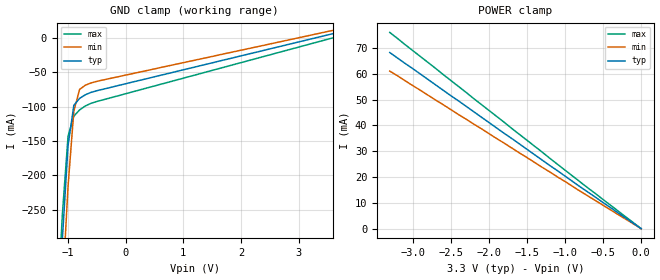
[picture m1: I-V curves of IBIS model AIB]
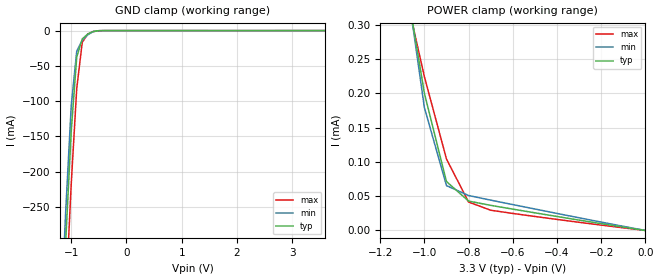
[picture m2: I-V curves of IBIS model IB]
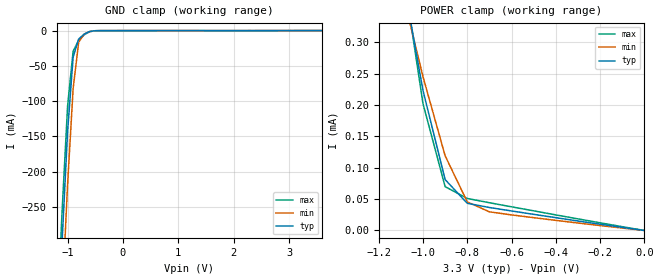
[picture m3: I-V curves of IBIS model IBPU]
|   Texas Instruments Incorporated
|   DVI group
|   IBIS Model for TFP401 Rev.st0n1
|   100 pin PowerPAD Package
[IBIS Ver]   4.0
[Comment char]   |_char
[File name]   tfp401n_st0.ibs
[File Rev]   1.0
[Date]   10/25/2002
[Source]   File originated at Texas Instruments Incorporated.
   Bus Solutions Department. All data based on SPICE
   simulation.
[Notes]   File created by Ellen Yeh.
   PIN #3 (ST) set to low.
|Revision log: 1.0, 10/25/2002 Original release
[Disclaimer]
(C) Copyright Texas Instruments Incorporated 2002
   All rights reserved
  Texas Instruments Incorporated hereby grants the user of this IBIS
model a non-exclusive, nontransferable license to use this IBIS model
under the following terms.  Before using this IBIS model, the user
should read this license.  If the user does not accept these terms,
the IBIS model should be returned to Texas Instruments within 30 days.
  The user is granted this license only to use the IBIS model and
is not granted rights to sell, load, rent, lease or license the IBIS
model in whole or in part, or in modified form to anyone other than
user.  User may modify the IBIS model to suit its specific applications
but rights to derivative works and such modifications shall belong to
Texas Instruments.
  This IBIS model is provided on an "AS IS" basis and Texas Instruments
makes absolutely no warranty with respect to the information contained
herein.  TEXAS INSTRUMENTS DISCLAIMS AND CUSTOMER WAIVES ALL WARRANTIES,
EXPRESS OR IMPLIED, INCLUDING WARRANTIES OF MERCHANTABILITY OR FITNESS
FOR A PARTICULAR PURPOSE. The entire risk as to quality and performance
is with the Customer. ACCORDINGLY, IN NO EVENT SHALL THE COMPANY BE LIABLE
FOR ANY DAMAGES, WHETHER IN CONTRACT OR TORT,INCLUDING ANY LOST PROFITS
OR OTHER INCIDENTAL, CONSEQUENTIAL, EXEMPLARY, OR PUNITIVE DAMAGES ARISING
OUT OF THE USE OR APPLICATION OF THE IBIS model provided in this package.
Further, Texas Instruments reserves the right to discontinue or make changes
without notice to any product herein to improve reliability, function, or
design. Texas Instruments does not convey any license under patent rights
or any other intellectual property rights, including those of third parties.
IBIS Open Forum disclaims all warranties. See DISCLAIM.TXT
in vhdl.org:/pub/IBIS/models for the full disclaimer.
[Copyright]   Copyright 2002, Texas Instruments, All Rights Reserved
[Component]   TFP401
[Manufacturer]  Texas Instruments Incorporated
[Package]
|   typ   min   max
R_pkg   0.051   0.049   0.054
L_pkg   2.9nH   2.7nH   3.2nH
C_pkg   0.44pF   0.36pF   0.5pF
[Pin]   signal_name   model_name   R_pin   L_pin   C_pin
1   DFO   IOBOD
2   PDZ   IBPU
3   ST   IB
4   PIXS   IB
5   GND   GND
6   DVDD   POWER
7   STAG   IB
8   SCDT   IOB
9   PDOZ   IBPU
10   QE0   OB
11   QE1   OB
12   QE2   OB
13   QE3   OB
14   QE4   OB
15   QE5   OB
16   QE6   OB
17   QE7   OB
18   OVDD   POWER
19   OGND   GND
20   QE8   OB
21   QE9   OB
22   QE10   OB
23   QE11   OB
24   QE12   OB
25   QE13   OB
26   QE14   OB
27   QE15   OB
28   OGND   GND
29   OVDD   POWER
30   QE16   OB
31   QE17   OB
32   QE18   OB
33   QE19   OB
34   QE20   OB
35   QE21   OB
36   QE22   OB
37   QE23   OB
38   DVDD   POWER
39   GND   GND
40   CTL1   IOB
41   CTL2   IOB
42   CTL3   IOB
43   OVDD   POWER
44   ODCK   OB2
45   OGND   GND
46   DE   OB
47   VSYNC   OB
48   HSYNC   OB
49   QO0   OB
50   QO1   OB
51   QO2   OB
52   QO3   OB
53   QO4   OB
54   QO5   OB
55   QO6   OB
56   QO7   OB
57   OVDD   POWER
58   OGND   GND
59   QO8   OB
60   QO9   OB
61   QO10   OB
62   QO11   OB
63   QO12   OB
64   QO13   OB
65   QO14   OB
66   QO15   OB
67   DVDD   POWER
68   GND   GND
69   QO16   OB
70   QO17   OB
71   QO18   OB
72   QO19   OB
73   QO20   OB
74   QO21   OB
75   QO22   OB
76   OGND   GND
77   QO23   OB
78   OVDD   POWER
79   AGND   GND
80   RX2+   AIB
81   RX2-   AIB
82   AVDD   POWER
83   AGND   GND
84   AVDD   POWER
85   RX1+   AIB
86   RX1-   AIB
87   AGND   GND
88   AVDD   POWER
89   AGND   GND
90   RX0+   AIB
91   RX0-   AIB
92   AGND   GND
93   RXC+   AIB
94   RXC-   AIB
95   AVDD   POWER
96   EXT_RES   AIB
97   PVDD   POWER
98   PGND   GND
99   RSVD   IBPU
100   OCK_INV   IB
| Models and submodels in the file (7): AIB (Input), IB (Input), IBPU (Input), IOB (I/O), IOBOD (I/O_open_sink), OB (3-state), OB2 (3-state)
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|   INPUT  MODEL
[Model]   AIB
Model_type   Input
Vinl = 2.85
Vinh = 3.0
| variable   typ   min   max
C_comp   2pF   NA   NA
|   typ   min   max
[Temperature Range]   25.0   70   0
[Voltage range]   3.3V   3.0V   3.6V
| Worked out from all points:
|   POWER clamp passes 1 mA (typ) near -0.05 V on its own axis
[GND_clamp]
|Voltage   I(typ)   I(min)   I(max)
-3.6V     -5.13A     -5.2A      -5.09A
-1.2V     -463mA     -543mA     -422mA
-1.1V     -295mA     -371mA     -259mA
-1V       -157mA     -216mA     -143mA
-900mV    -98.3mA    -107mA     -114mA
-800mV    -88.2mA    -75.2mA    -105mA
-700mV    -82.9mA    -69mA      -99.2mA
-500mV    -77mA      -63.4mA    -92.7mA
3.6V      6.08mA     10.9mA     8.48pA
[Power_clamp]
|Note that the [Power_clamp] voltage table is referenced to Vcc
|and is calculated using Vtable=Vcc-Vmeasured.
|Voltage   I(typ)   I(min)   I(max)
-3.3V     68.3mA     61.1mA     76.1mA
-1.2V     24.5mA     22mA       27.3mA
-800mV    16.2mA     14.5mA     18.1mA
0V        10.1pA     47.9pA     8.48pA
|   INPUT  MODEL
[Model]   IB
Model_type   Input
Vinl = 0.8
Vinh = 2.0
| variable   typ   min   max
C_comp   2pF   NA   NA
|   typ   min   max
[Temperature Range]   25.0   70   0
[Voltage range]   3.3V   3.0V   3.6V
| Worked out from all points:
|   GND clamp passes 1 mA (typ) near -0.58 V on its own axis
|   POWER clamp passes 1 mA (typ) near -1.37 V on its own axis
[GND_clamp]
|Voltage   I(typ)   I(min)   I(max)
-3.6V     -5.15A     -5.11A     -5.23A
-1.2V     -475mA     -430mA     -560mA
-1.1V     -300mA     -257mA     -383mA
-1V       -143mA     -107mA     -218mA
-900mV    -37.5mA    -29.1mA    -82.2mA
-800mV    -11.8mA    -13.8mA    -16.6mA
-700mV    -4.88mA    -5.9mA     -4.87mA
-600mV    -1.21mA    -1.39mA    -1.38mA
-500mV    -134uA     -137uA     -206uA
3.6V      15.1uA     34.3pA     24.8uA
[Power_clamp]
|Note that the [Power_clamp] voltage table is referenced to Vcc
|and is calculated using Vtable=Vcc-Vmeasured.
|Voltage   I(typ)   I(min)   I(max)
-3.3V     5.59mA     6.88mA     4.02mA
-1.1V     393uA      406uA      367uA
-1V       200uA      179uA      224uA
-900mV    71.2uA     65.3uA     104uA
-800mV    42.8uA     50.9uA     41.4uA
-700mV    36.6uA     44.2uA     29.5uA
0V        35.3pA     34.3pA     99.7pA
|   INPUT  MODEL WITH PULL UP
[Model]   IBPU
Model_type   Input
Vinl = 0.8
Vinh = 2.0
| variable   typ   min   max
C_comp   2pF   NA   NA
|   typ   min   max
[Temperature Range]   25.0   70   0
[Voltage range]   3.3V   3.0V   3.6V
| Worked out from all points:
|   GND clamp passes 1 mA (typ) near -0.58 V on its own axis
|   POWER clamp passes 1 mA (typ) near -1.36 V on its own axis
[GND_clamp]
|Voltage   I(typ)   I(min)   I(max)
-3.6V     -5.15A     -5.23A     -5.11A
-1.2V     -475mA     -560mA     -430mA
-1.1V     -300mA     -383mA     -257mA
-1V       -143mA     -218mA     -107mA
-900mV    -37.5mA    -82.2mA    -29.2mA
-800mV    -11.9mA    -16.6mA    -13.9mA
-700mV    -4.91mA    -4.9mA     -5.95mA
-600mV    -1.25mA    -1.4mA     -1.45mA
-500mV    -184uA     -239uA     -206uA
3.6V      15.1uA     24.8uA     34.3pA
[Power_clamp]
|Note that the [Power_clamp] voltage table is referenced to Vcc
|and is calculated using Vtable=Vcc-Vmeasured.
|Voltage   I(typ)   I(min)   I(max)
-3.3V     5.62mA     4.04mA     6.91mA
-1.1V     420uA      390uA      436uA
-1V       223uA      245uA      202uA
-900mV    81.1uA     119uA      69.8uA
-800mV    43.3uA     45.5uA     51uA
-700mV    36.6uA     29.7uA     44.2uA
0V        35.3pA     99.7pA     34.3pA
